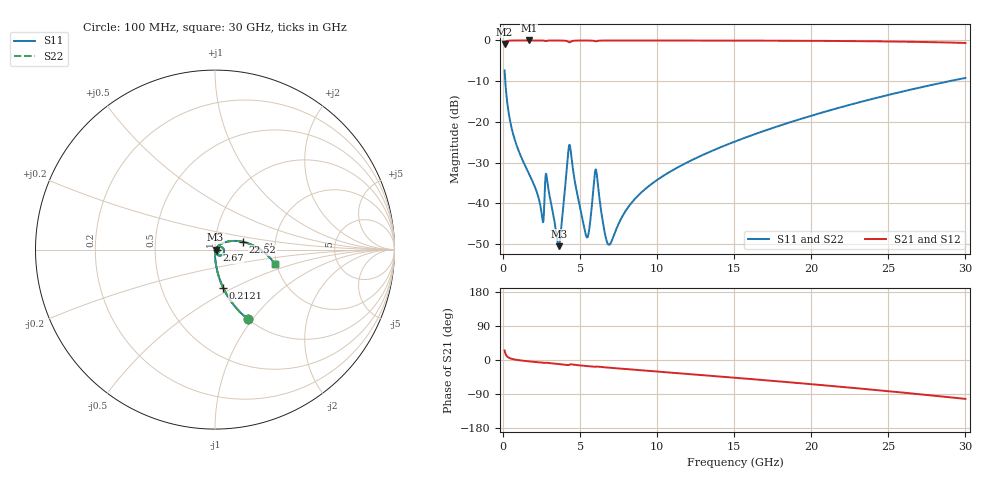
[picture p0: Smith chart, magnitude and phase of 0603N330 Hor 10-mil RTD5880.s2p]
# GHz S MA R 50
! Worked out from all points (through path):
!   3201 points, 100 MHz to 30 GHz, reference 50 ohm
!   highest |S21| = -0.01 dB at 1.688 GHz (marker M1); lowest = -0.9 dB at 100 MHz (marker M2)
!   group delay of S21, straight-line fit = 9.58 ps
!   lowest |S11| = -50.5 dB at 3.613 GHz (marker M3), VSWR 1.01, Z = 50.3 - j0.0947 ohm
!   |S11| at or under -10 dB: 142.8 MHz to 28.96 GHz (28.82 GHz wide, 198 % of centre)
!   |S22| runs from -50.5 to -7.3 dB; largest |S21 - S12| = 0
!   S11 on the Smith chart (normalised r, x): 100 MHz: 1.00, -0.95; 212.1 MHz: 1.00, -0.45; 2.67 GHz: 1.02, -0.00; 22.52 GHz: 1.37, +0.12; 30 GHz: 1.97, -0.37
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0.1  0.4299 -64.8  0.9025 25.2  0.9025 25.2  0.4299 -64.8
0.212125  0.2186 -77.9  0.9754 12.0  0.9754 12.0  0.2186 -77.9
0.6793125  0.06809 -87.5  0.9969 1.9  0.9969 1.9  0.06809 -87.5
1.688438  0.02299 -90.8  0.9985 -3.7  0.9985 -3.7  0.02299 -90.8
2.510687  0.007286 -74.0  0.9971 -7.0  0.9971 -7.0  0.007286 -74.0
2.669531  0.009291 -11.1  0.9907 -7.9  0.9907 -7.9  0.009291 -11.1
2.875094  0.01843 -71.5  0.9917 -7.6  0.9917 -7.6  0.01843 -71.5
3.61325  0.002993 -18.3  0.997 -10.7  0.997 -10.7  0.002993 -18.3
3.753406  0.004566 26.2  0.9963 -11.2  0.9963 -11.2  0.004566 26.2
4.304688  0.05236 -16.2  0.9477 -12.5  0.9477 -12.5  0.05236 -16.2
5.089563  0.007405 -73.4  0.9961 -14.7  0.9961 -14.7  0.007405 -73.4
5.500687  0.003936 -12.1  0.996 -16.2  0.996 -16.2  0.003936 -12.1
6.033281  0.02577 -29.6  0.9747 -17.5  0.9747 -17.5  0.02577 -29.6
6.593906  0.004409 -54.2  0.9963 -19.3  0.9963 -19.3  0.004409 -54.2
6.911594  0.003135 -7.3  0.9968 -20.4  0.9968 -20.4  0.003135 -7.3
8.201031  0.009448 48.2  0.9971 -24.6  0.9971 -24.6  0.009448 48.2
10.06978  0.01986 50.8  0.9967 -30.6  0.9967 -30.6  0.01986 50.8
15.05  0.05753 39.5  0.9944 -46.8  0.9944 -46.8  0.05753 39.5
20.03956  0.1197 23.9  0.988 -63.9  0.988 -63.9  0.1197 23.9
22.525  0.1627 15.3  0.9813 -72.9  0.9813 -72.9  0.1627 15.3
25.01978  0.2149 6.1  0.9707 -82.4  0.9707 -82.4  0.2149 6.1
30  0.3464 -13.8  0.9309 -102.6  0.9309 -102.6  0.3464 -13.8
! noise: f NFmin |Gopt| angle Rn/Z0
0.1  0.0002944  0.919  0.3934  0.0008033
3.417  0.004402  0.8244  10.1  0.005226
6.743  0.006926  0.7858  19.85  0.006451
10.06  0.008063  0.7357  29.39  0.005712
13.39  0.00998  0.7216  38.74  0.006345
16.7  0.01193  0.7149  47.81  0.006944
20.03  0.01396  0.7128  56.63  0.007486
23.35  0.01608  0.7141  65.12  0.007974
26.67  0.01835  0.7183  73.33  0.008416
30  0.02083  0.7248  81.25  0.008818
